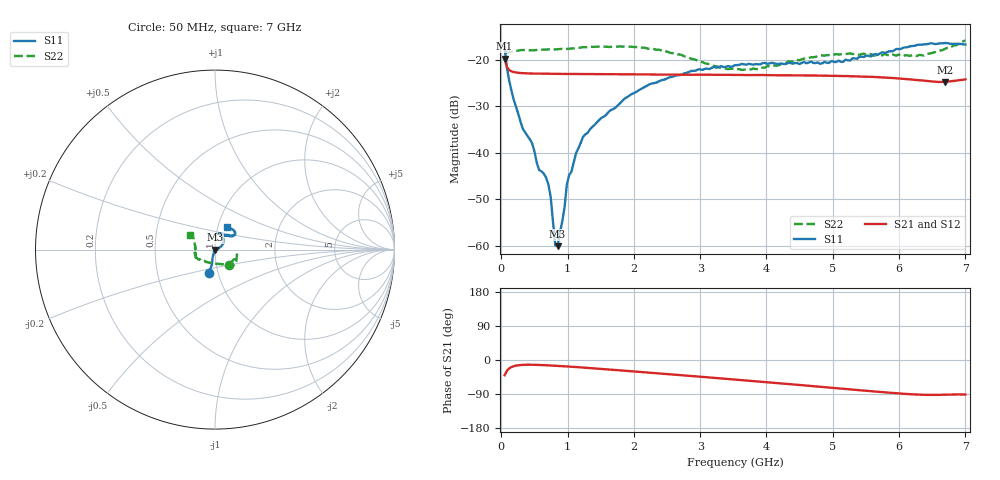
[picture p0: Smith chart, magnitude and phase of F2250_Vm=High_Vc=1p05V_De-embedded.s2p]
! Integrated Device Technology
! Corporate Headquarters
! 6024 Silver Creek Valley Road
! San Jose, CA 95138  USA
! Phone:  1-408-284-8200
! Toll Free:  1-800-223-1366
! Webpage:  http://www.idt.com/
! Timing and RF Division
! 515 Groton Road, Suite 102
! Westford, MA 01886-6024
! Device:  F2250
! Description: Voltage Variable RF Attenuator
! Frequency:  50.0 -  6000.00 MHz
! Package:  3x3 mm Thin QFN Plastic Package: 16 pin
! Ports:  2 RF, 3 DC
!  Pin  1  = GND
!  Pin  2  = NC
!  Pin  3  = RF1  = Port 1
!  Pin  4  = NC
!  Pin  5  = GND
!  Pin  6  = GND
!  Pin  7  = GND
!  Pin  8  = GND
!  Pin  9  = NC
!  Pin 10  = RF2  = Port 2
!  Pin 11  = NC
!  Pin 12  = GND
!  Pin 13  = GND
!  Pin 14  = VCNTRL
!  Pin 15  = VDD
!  Pin 16  = VMODE
! Vcntrl:  1.050 Volts
! Vmode:  +3.300 Volts
! Vdd:  +3.30  Volts
! Current:  1.328 mA
! Data:  The device was measured on a the F2250 evaluation board which has
!  individual transmission lines to the RF pins.  Data was collected
!  using a calibrated network analyzer.  The evaluation board was
!  de-embedded using a TRL calibration technique.
!  The reference plane is the edge of the package pin.
! Misc:  SN 10
!  Action Tracker AT0258
! Date Measured:  2014-11-26
! Date:  2015-10-15  MJV
! Note:
!  Integrated Device Technology supplies this data as a sample of measured
!  data at the package pin for this product.  Your particular data for this
!  product may vary.
!  Data was taken at 25 degrees C.
!  Integrated Device Technology reserves the right to change this data at anytime.
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# GHz S dB R 50
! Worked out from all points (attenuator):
!   201 points, 50 MHz to 7 GHz, reference 50 ohm
!   highest |S21| = -19.80 dB at 50 MHz (marker M1); lowest = -24.8 dB at 6.687 GHz (marker M2)
!   lowest |S11| = -60.1 dB at 849.2 MHz (marker M3), VSWR 1.00, Z = 50 - j0.0982 ohm
!   |S11| at or under -10 dB: start of sweep to end of sweep
!   |S22| runs from -22.2 to -15.9 dB; largest |S21 - S12| = 0.00029
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0.05  -17.34 -104.6  -19.80 -40.3  -19.80 -40.3  -18.82 -47.5
0.1195  -24.58 -104.1  -22.27 -22.2  -22.26 -22.1  -18.36 -18.0
0.29325  -33.52 -107.5  -22.91 -13.2  -22.91 -13.2  -17.97 -13.4
0.467  -38.09 -118.9  -23.01 -12.5  -23.00 -12.5  -18.03 -14.0
0.57125  -43.76 -120.6  -23.03 -13.1  -23.02 -13.1  -17.94 -16.2
0.64075  -44.54 -117.6  -23.05 -13.6  -23.05 -13.5  -17.84 -17.1
0.71025  -46.88 -112.1  -23.08 -14.1  -23.06 -14.2  -17.82 -18.9
0.745  -49.54 -109.8  -23.08 -14.5  -23.06 -14.5  -17.81 -19.4
0.8145  -59.94 -129.3  -23.09 -15.1  -23.08 -15.1  -17.83 -21.1
0.84925  -60.14 -92.7  -23.09 -15.5  -23.08 -15.5  -17.80 -22.2
0.9535  -51.86 -42.9  -23.10 -16.6  -23.09 -16.6  -17.79 -24.2
0.98825  -46.94 -23.6  -23.11 -17.0  -23.10 -17.0  -17.74 -24.8
1.12725  -40.15 4.1  -23.12 -18.6  -23.11 -18.6  -17.52 -26.9
1.2315  -36.67 9.7  -23.12 -19.9  -23.11 -19.9  -17.34 -29.0
1.857  -28.44 27.2  -23.16 -28.3  -23.17 -28.3  -17.20 -36.7
2.37825  -24.69 38.7  -23.24 -35.3  -23.23 -35.4  -17.89 -43.2
3.525  -21.20 68.0  -23.30 -51.6  -23.31 -51.7  -22.09 -91.8
4.7065  -20.73 70.1  -23.43 -69.1  -23.43 -69.1  -19.51 -149.1
5.85325  -18.20 38.6  -23.95 -86.3  -23.93 -86.4  -19.12 -171.1
6.3745  -16.74 39.6  -24.54 -91.9  -24.53 -92.0  -19.14 169.8
6.68725  -16.46 46.7  -24.82 -91.3  -24.80 -91.5  -17.74 154.3
7  -16.78 61.9  -24.25 -91.2  -24.24 -91.4  -15.90 148.6
